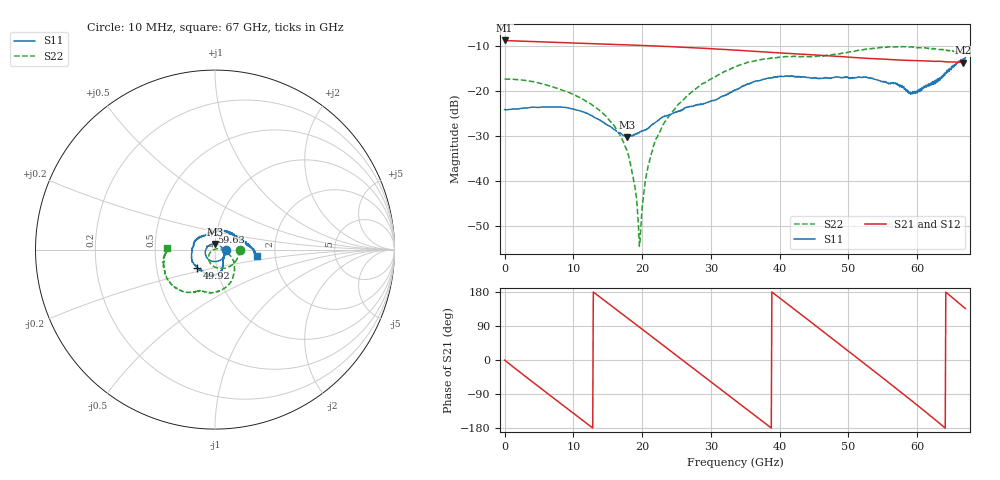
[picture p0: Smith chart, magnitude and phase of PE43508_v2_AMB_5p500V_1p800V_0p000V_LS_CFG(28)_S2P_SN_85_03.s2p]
!Keysight Technologies,N5227A,US51270237,A.10.43.00
!Date: Wednesday, August 22, 2018 17:09:28
!Correction: S11(Full 2 Port(1,3))
!S31(Full 2 Port(1,3))
!S13(Full 2 Port(1,3))
!S33(Full 2 Port(1,3))
!S2P File: Measurements: S11, S31, S13, S33:
# Hz S  dB  R 50
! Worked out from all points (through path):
!   801 points, 10 MHz to 67 GHz, reference 50 ohm
!   highest |S21| = -8.73 dB at 10 MHz (marker M1); lowest = -13.7 dB at 66.67 GHz (marker M2)
!   group delay of S21, straight-line fit = 38.8 ps
!   lowest |S11| = -30.2 dB at 17.76 GHz (marker M3), VSWR 1.06, Z = 49.8 + j3.07 ohm
!   |S11| at or under -10 dB: start of sweep to end of sweep
!   |S22| runs from -54.5 to -10.1 dB; largest |S21 - S12| = 0.0022
!   S11 on the Smith chart (normalised r, x): 10 MHz: 1.13, -0.00; 49.92 GHz: 0.80, -0.17; 59.63 GHz: 0.94, +0.19; 67 GHz: 1.61, -0.12
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1e7  -24.10 -0.6  -8.73 -0.2  -8.74 -0.2  -17.29 -0.4
5.70415e9  -23.53 -84.9  -9.06 -80.8  -9.06 -80.7  -18.46 -59.3
8.300012e9  -23.55 -118.5  -9.21 -116.9  -9.20 -116.8  -19.75 -83.1
1.123082e10  -24.55 -154.1  -9.37 -157.5  -9.37 -157.4  -21.65 -106.7
1.558518e10  -28.11 141.3  -9.60 142.4  -9.60 142.4  -27.08 -139.1
1.776235e10  -30.25 91.1  -9.72 112.3  -9.72 112.3  -33.09 -156.7
1.87672e10  -29.70 65.1  -9.78 98.4  -9.77 98.4  -39.85 -172.2
1.94371e10  -29.32 50.7  -9.81 89.1  -9.82 89.1  -49.16 164.9
1.968831e10  -29.05 44.7  -9.83 85.6  -9.83 85.6  -53.58 90.5
2.07769e10  -28.39 22.7  -9.90 70.5  -9.90 70.5  -37.49 21.9
2.236791e10  -26.48 -4.8  -10.00 48.5  -10.00 48.5  -29.70 4.5
2.722469e10  -23.43 -45.7  -10.34 -19.0  -10.33 -18.9  -20.17 -24.0
3.049045e10  -22.01 -55.5  -10.61 -64.4  -10.60 -64.4  -16.91 -40.7
3.3505e10  -19.78 -64.8  -10.88 -106.3  -10.88 -106.3  -14.62 -57.8
3.88642e10  -17.09 -91.3  -11.39 179.4  -11.40 179.4  -12.65 -85.7
4.472582e10  -17.10 -118.2  -11.91 97.5  -11.90 97.6  -12.34 -107.3
4.991755e10  -16.95 -134.8  -12.43 24.3  -12.43 24.3  -11.36 -118.3
5.586291e10  -18.42 169.5  -12.95 -59.8  -12.95 -60.1  -10.16 -140.4
5.96311e10  -20.05 101.7  -13.21 -113.8  -13.23 -114.0  -10.31 -155.1
6.331555e10  -17.57 32.0  -13.37 -168.4  -13.42 -168.6  -10.75 -169.7
6.666505e10  -13.21 -5.4  -13.66 140.9  -13.72 141.1  -11.48 179.9
6.7e10  -12.50 -8.5  -13.65 135.7  -13.71 135.9  -11.54 177.8
